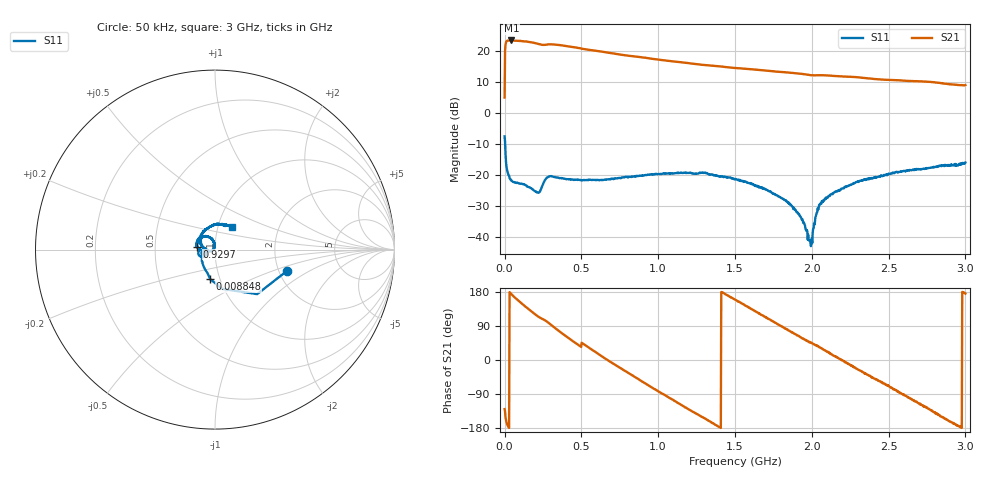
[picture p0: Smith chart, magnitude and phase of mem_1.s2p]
! NanoVNA-App
! Date: 2024-02-22 10:33:23
! Start: 50kHz Stop: 3.0001GHz Points: 1024
! S-Parameter data: F S11 S21 S12 S22
# Hz S RI R 50
!  Frequency  S11_Real  S11_Imag  S21_Real  S21_Imag  S12_Real  S12_Imag  S22_Real  S22_Imag
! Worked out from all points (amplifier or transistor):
!   1024 points, 50 kHz to 3 GHz, reference 50 ohm
!   highest |S21| = 23.4 dB at 44.04 MHz (marker M1)
!   |S21| within 3 dB of that: 3.475 MHz to 548.3 MHz (544.8 MHz wide, 197 % of centre)
!   S11 on the Smith chart (normalised r, x): 50 kHz: 2.23, -0.63; 8.848 MHz: 0.90, -0.30; 929.7 MHz: 0.82, +0.03; 3 GHz: 1.17, +0.31
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50000  0.4035 -0.1169  -1.133 -1.37  0 0  0 0
8847654  -0.0269 -0.1646  -12.63 -5.011  0 0  0 0
2.057786e7  -0.0659 -0.0868  -14.54 -1.668  0 0  0 0
4.403827e7  -0.0743 -0.0372  -14.66 1.627  0 0  0 0
1.056218e8  -0.0722 -0.00897  -12.61 7.012  0 0  0 0
1.642729e8  -0.0631 -0.00476  -9.19 10.38  0 0  0 0
2.903726e8  -0.0907 -0.029  -1.495 12.69  0 0  0 0
4.135397e8  -0.0861 -0.000654  6.149 10.13  0 0  0 0
4.83921e8  -0.084 0.000954  8.679 6.958  0 0  0 0
5.015163e8  -0.0832 0.000823  7.611 7.749  0 0  0 0
6.891996e8  -0.0868 0.00238  9.217 -0.7995  0 0  0 0
8.152993e8  -0.0933 0.00641  6.688 -4.97  0 0  0 0
9.296688e8  -0.1 0.0169  3.242 -6.95  0 0  0 0
1.00005e9  -0.1009 0.025  0.9214 -7.187  0 0  0 0
1.246384e9  -0.0904 0.0559  -4.767 -3.875  0 0  0 0
1.501516e9  -0.0448 0.0733  -4.965 1.889  0 0  0 0
1.741985e9  -0.0106 0.0504  -1.089 4.597  0 0  0 0
2.00005e9  -0.00947 0.000543  2.899 2.832  0 0  0 0
2.231722e9  -0.0655 0.011  3.8 -0.6189  0 0  0 0
2.501516e9  -0.0786 0.0676  1.216 -3.206  0 0  0 0
2.791839e9  -0.0193 0.1328  -2.271 -2.158  0 0  0 0
3.00005e9  0.0946 0.1283  -2.807 0.2357  0 0  0 0
